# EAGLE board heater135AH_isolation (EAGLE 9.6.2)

Size 173.6 x 175 mm. Coordinates in mm from the lower left corner, seen from the top.
Outline: 0,0 0,175 71.8,175 71.8,165 101.8,165 101.8,175 173.6,175 173.6,0 0,0
Copper layers (1*16): Top 0.035mm / dielectric 1.5mm / Bottom 0.035mm
Design rules "default": minimum track width 6mil, minimum drill 0.35mm, track to track 6mil, track to pad 6mil, pad to pad 6mil, via to via 6mil, smd to smd 6mil, copper to edge 40mil, drill to drill 6mil, minimum pad ring 10mil, minimum via ring 8mil, stop-mask expansion 4mil, vias tented up to drill 0mil, thermal gap 10mil

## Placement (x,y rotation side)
U$1  [CE-4MM]  0.84,159.13 0 top

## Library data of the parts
U$1 = logo

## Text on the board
tPlace: ECS, Am Wenigerflur 14, 54498 Piesport | HEATER280_304 | ISOLATION PLATE / (END PLATE)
